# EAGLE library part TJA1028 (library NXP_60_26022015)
LIN transceiver with integrated voltage regulator The TJA1028 is a LIN 2.0/2.1/SAE J2602 transceiver with an integrated low-drop voltage regulator. The voltage regulator can deliver up to 70 mA and is available in 3.3 V and 5.0 V variants. TJA1028 facilitates the development of compact nodes in Local Interconnect Network (LIN) bus systems. To support robust designs, the TJA1028 offers strong ElectroStatic Discharge (ESD) performance and can withstand high voltages on the LIN bus. In order to minimize current consumption, the TJA1028 supports a Sleep mode in which the LIN transceiver and the voltage regulator are powered down while still having wake-up capability via the LIN bus. The TJA1028 comes in an SO8 package, and also in a 3 mm  3 mm HVSON8 package that reduces the required board space by over 70 %. This feature can prove extremely valuable when board space is limited. AAL Eindhoven MK
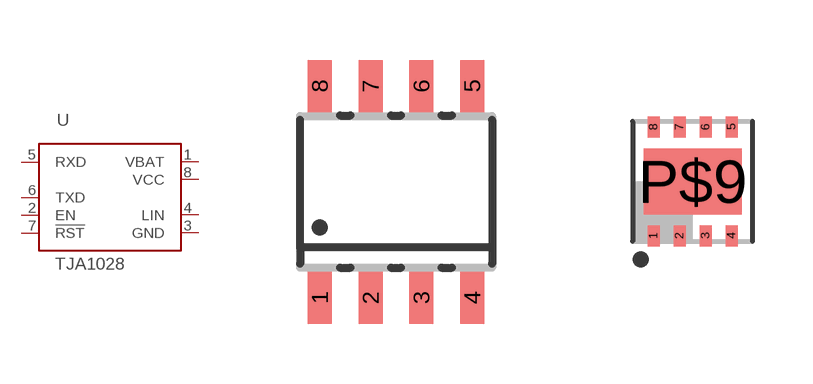
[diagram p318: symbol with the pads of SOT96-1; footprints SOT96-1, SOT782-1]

Designator prefix U

## TJA1028T  [SOT96-1]
1  VBAT  pwr
2  EN  in
3  GND  pwr
4  LIN  in
5  RXD  in
6  TXD  out
7  !RST  out
8  VCC  pwr

## TJA1028TK  [SOT782-1]
Pads as for SOT96-1

## Footprint SOT96-1 (pad centres in mm)
SOT96-1 SO8: plastic small outline package; 8 leads; body width 3.9 mm JEDEC: MS-012 IEC: 076E03
smd 0.6 x 1.3: 1 -1.905,-2.65; 2 -0.635,-2.65; 3 0.635,-2.65; 4 1.905,-2.65; 5 1.905,2.65; 6 0.635,2.65; 7 -0.635,2.65; 8 -1.905,2.65

## Footprint SOT782-1 (pad centres in mm)
SOT782-1 HVSON8: plastic thermal enhanced very thin small outline package; no leads; 8 terminals; body 3 x 3 x 0.85 mm JEDEC: MO-229 IEC: -- JEITA: --
smd 0.3 x 0.525: 1 -0.975,-1.363; 2 -0.325,-1.363; 3 0.325,-1.363; 4 0.975,-1.363; 5 0.975,1.363; 6 0.325,1.363; 7 -0.325,1.363; 8 -0.975,1.363
smd 2.45 x 1.65: P$9 0,0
